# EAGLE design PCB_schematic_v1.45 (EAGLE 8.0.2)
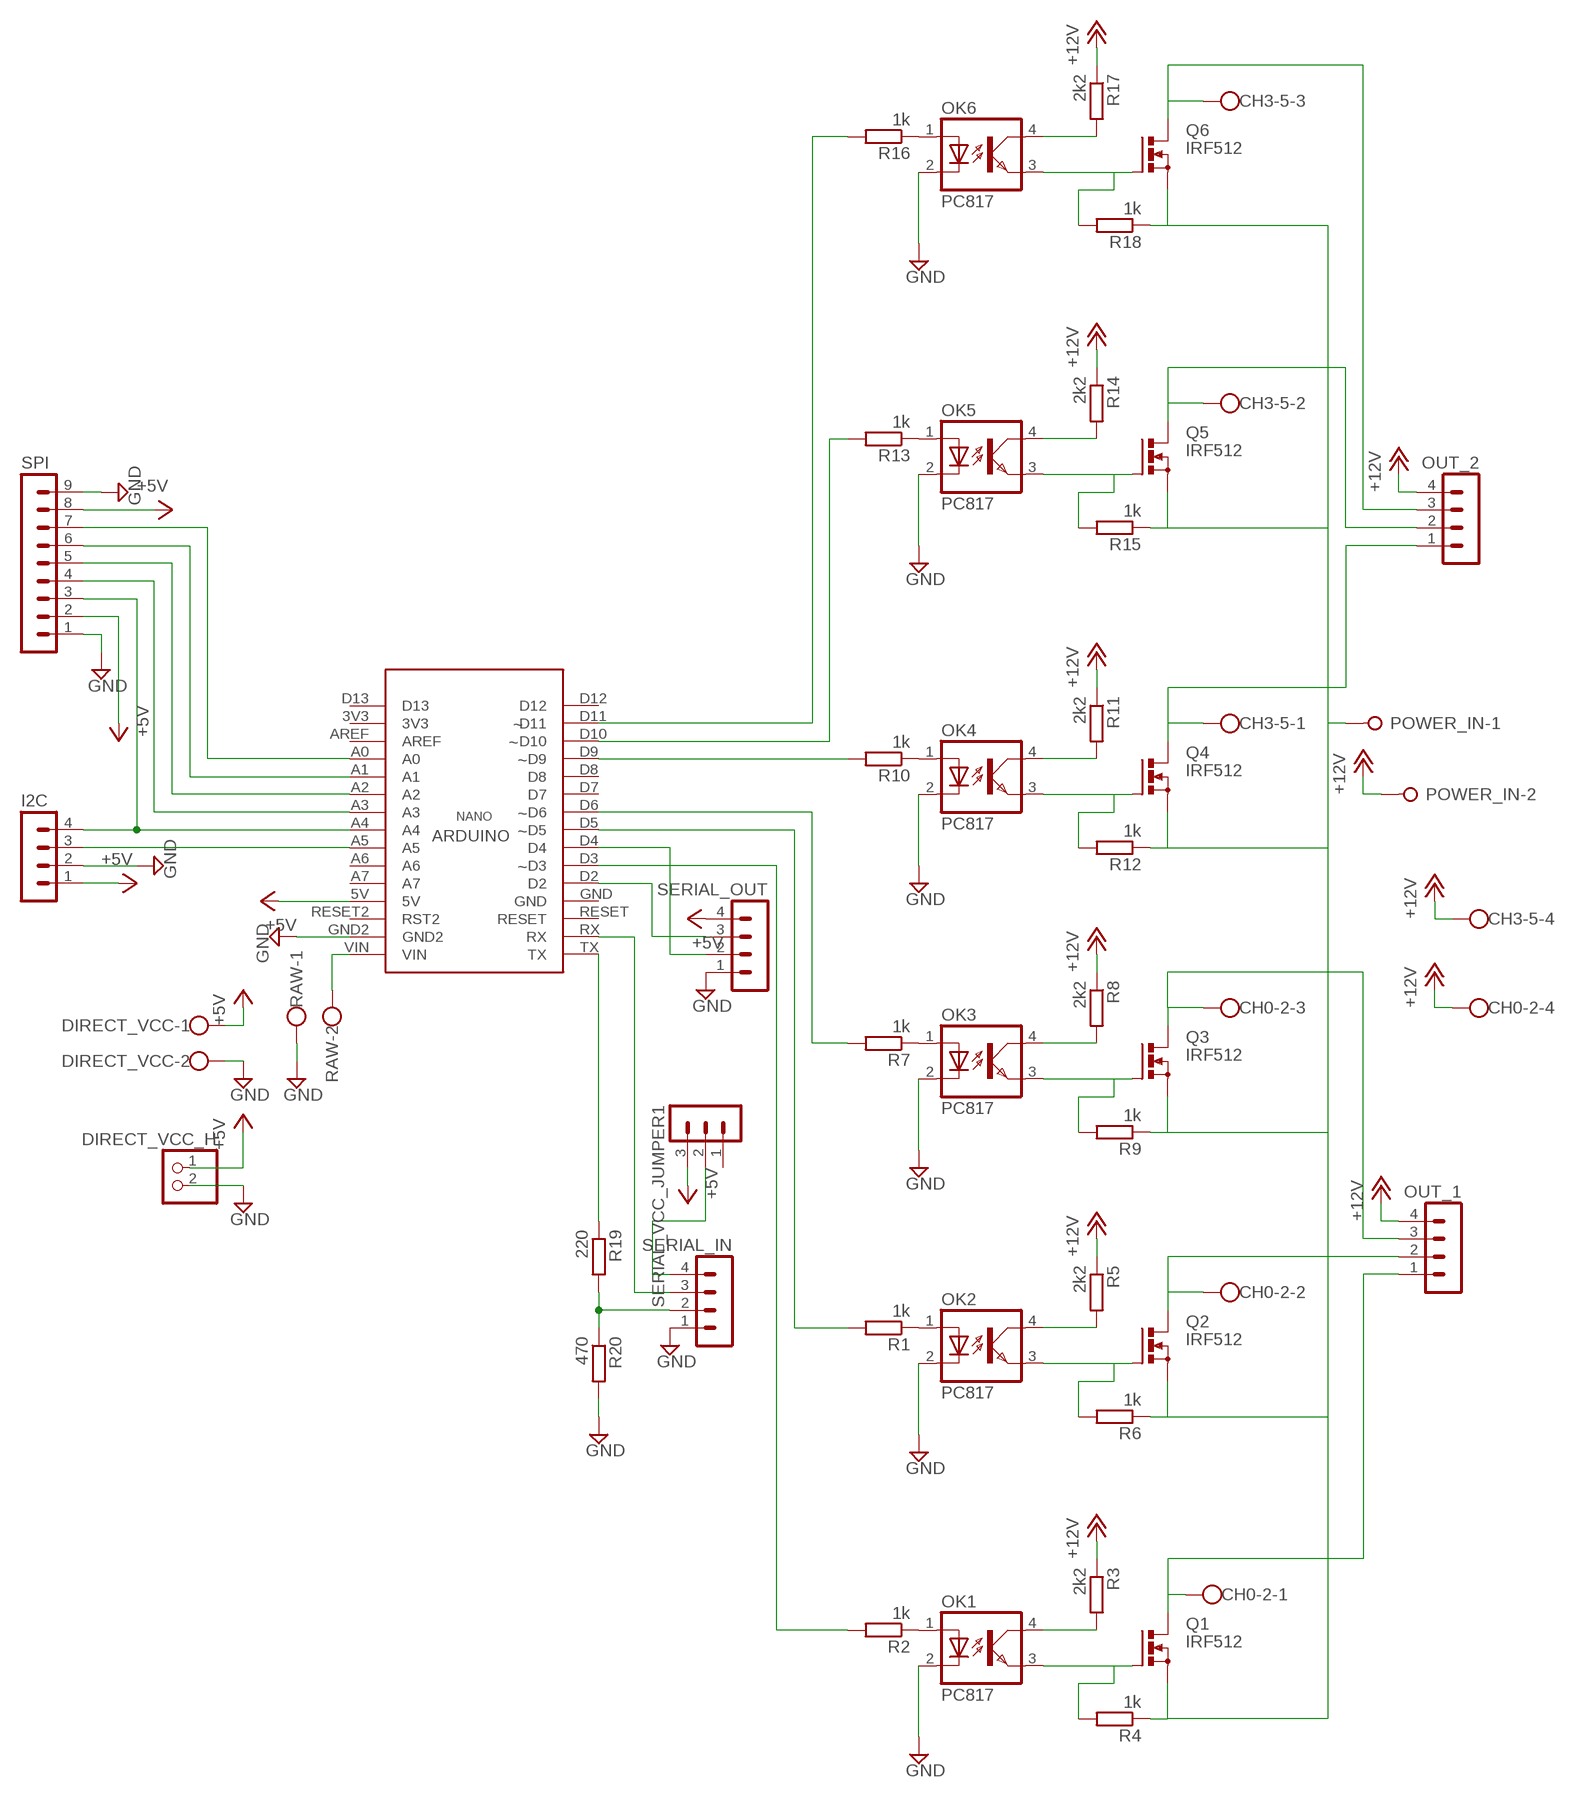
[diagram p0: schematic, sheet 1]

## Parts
CH0-2  W237-4  [W237-4]
CH3-5  W237-4  [W237-4]
DIRECT_VCC  W237-102  [W237-102]
DIRECT_VCC_H  PINHD-1X2  [1X02]
I2C  MA04-1  [MA04-1]
OK1  PC817  [DIL04]
OK2  PC817  [DIL04]
OK3  PC817  [DIL04]
OK4  PC817  [DIL04]
OK5  PC817  [DIL04]
OK6  PC817  [DIL04]
OUT_1  MA04-1  [MA04-1]
OUT_2  MA04-1  [MA04-1]
POWER_IN  W237-02P  [W237-132]
Q1  IRF512  [TO220BV]
Q2  IRF512  [TO220BV]
Q3  IRF512  [TO220BV]
Q4  IRF512  [TO220BV]
Q5  IRF512  [TO220BV]
Q6  IRF512  [TO220BV]
R1  1k  R-EU_0207/10  [0207/10]
R2  1k  R-EU_0207/10  [0207/10]
R3  2k2  R-EU_0207/10  [0207/10]
R4  1k  R-EU_0207/10  [0207/10]
R5  2k2  R-EU_0207/10  [0207/10]
R6  1k  R-EU_0207/10  [0207/10]
R7  1k  R-EU_0207/10  [0207/10]
R8  2k2  R-EU_0207/10  [0207/10]
R9  1k  R-EU_0207/10  [0207/10]
R10  1k  R-EU_0207/10  [0207/10]
R11  2k2  R-EU_0207/10  [0207/10]
R12  1k  R-EU_0207/10  [0207/10]
R13  1k  R-EU_0207/10  [0207/10]
R14  2k2  R-EU_0207/10  [0207/10]
R15  1k  R-EU_0207/10  [0207/10]
R16  1k  R-EU_0207/10  [0207/10]
R17  2k2  R-EU_0207/10  [0207/10]
R18  1k  R-EU_0207/10  [0207/10]
R19  220  R-EU_0207/10  [0207/10]
R20  470  R-EU_0207/10  [0207/10]
RAW  W237-102  [W237-102]
SERIAL_IN  MA04-1  [MA04-1]
SERIAL_OUT  MA04-1  [MA04-1]
SERIAL_VCC_JUMPER1  MA03-1  [MA03-1]
SPI  MA09-1  [MA09-1]
U$2  NANO  [NANO]

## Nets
+5V: DIRECT_VCC.1 DIRECT_VCC_H.1 I2C.1 SERIAL_OUT.4 SERIAL_VCC_JUMPER1.3 SPI.2 SPI.8 U$2.5V
+12V: CH0-2.4 CH3-5.4 OUT_1.4 OUT_2.4 POWER_IN.2 R3.1 R5.1 R8.1 R11.1 R14.1 R17.1
CS: SPI.7 U$2.A0
D1: SPI.4 U$2.A3
DC: SPI.6 U$2.A1
EXT_GND: POWER_IN.1 Q1.S Q2.S Q3.S Q4.S Q5.S Q6.S R4.1 R6.1 R9.1 R12.1 R15.1 R18.1
FET0_GATE: OK1.3(EMIT) Q1.G R4.2
FET0_GATE1: OK2.3(EMIT) Q2.G R6.2
FET0_GATE2: OK3.3(EMIT) Q3.G R9.2
FET0_GATE3: OK4.3(EMIT) Q4.G R12.2
FET0_GATE4: OK5.3(EMIT) Q5.G R15.2
FET0_GATE5: OK6.3(EMIT) Q6.G R18.2
GND: DIRECT_VCC.2 DIRECT_VCC_H.2 I2C.2 OK1.2(C) OK2.2(C) OK3.2(C) OK4.2(C) OK5.2(C) OK6.2(C) R20.2 RAW.1 SERIAL_IN.1 SERIAL_OUT.1 SPI.1 SPI.9 U$2.GND2
IC_PWM_OUT_0: R2.2 U$2.D3
IC_PWM_OUT_0_BASE: OK1.1(A) R2.1
IC_PWM_OUT_0_BASE1: OK2.1(A) R1.1
IC_PWM_OUT_0_BASE2: OK3.1(A) R7.1
IC_PWM_OUT_0_BASE3: OK4.1(A) R10.1
IC_PWM_OUT_0_BASE4: OK5.1(A) R13.1
IC_PWM_OUT_0_BASE5: OK6.1(A) R16.1
IC_PWM_OUT_1: R1.2 U$2.D5
IC_PWM_OUT_2: R7.2 U$2.D6
IC_PWM_OUT_3: R10.2 U$2.D9
IC_PWM_OUT_4: R13.2 U$2.D10
IC_PWM_OUT_5: R16.2 U$2.D11
N$1: OK1.4(COL) R3.2
N$3: OK2.4(COL) R5.2
N$5: OK3.4(COL) R8.2
N$7: OK4.4(COL) R11.2
N$9: OK5.4(COL) R14.2
N$11: OK6.4(COL) R17.2
OLED_RES: SPI.5 U$2.A2
OUT_RX: SERIAL_OUT.3 U$2.D2
OUT_TX: SERIAL_OUT.2 U$2.D4
OUTPUT_0: CH0-2.1 OUT_1.1 Q1.D
OUTPUT_1: CH0-2.2 OUT_1.2 Q2.D
OUTPUT_2: CH0-2.3 OUT_1.3 Q3.D
OUTPUT_3: CH3-5.1 OUT_2.1 Q4.D
OUTPUT_4: CH3-5.2 OUT_2.2 Q5.D
OUTPUT_5: CH3-5.3 OUT_2.3 Q6.D
RAW_INPUT: RAW.2 U$2.VIN
RX: SERIAL_IN.3 U$2.RX
SCL: I2C.3 U$2.A5
SDA_/_D0: I2C.4 SPI.3 U$2.A4
SERIAL_VCC: SERIAL_IN.4 SERIAL_VCC_JUMPER1.2
TX_3,3V: R19.2 R20.1 SERIAL_IN.2
TX_5V: R19.1 U$2.TX
Unconnected: SERIAL_VCC_JUMPER1.1 U$2.3V3 U$2.A6 U$2.A7 U$2.AREF U$2.D7 U$2.D8 U$2.D12 U$2.D13 U$2.GND U$2.RESET U$2.RESET2(RST2)

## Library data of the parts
CH0-2 CH3-5 = con-wago-500:W237-4: WAGO SCREW CLAMP; OC_FARNELL: unknown; OC_NEWARK: unknown
DIRECT_VCC RAW = con-wago-500:W237-102: WAGO SCREW CLAMP; MPN: 237-102; OC_FARNELL: unknown; OC_NEWARK: 70K9898
DIRECT_VCC_H = pinhead:PINHD-1X2: PIN HEADER
I2C OUT_1 OUT_2 SERIAL_IN SERIAL_OUT = con-lstb:MA04-1: PIN HEADER; OC_FARNELL: unknown; OC_NEWARK: unknown
OK1-OK6 = optocoupler:PC817: SHARP OPTO COUPLER; MPN: PC817X4J000F; OC_FARNELL: 9707727; OC_NEWARK: 97K7059
POWER_IN = con-wago-508:W237-02P: WAGO SREW CLAMP; OC_FARNELL: unknown; OC_NEWARK: unknown
Q1-Q6 = transistor-power:IRF512: N-CHANNEL MOS FET
R1-R20 = rcl:R-EU_: RESISTOR, European symbol
SERIAL_VCC_JUMPER1 = con-lstb:MA03-1: PIN HEADER; OC_FARNELL: unknown; OC_NEWARK: unknown
SPI = con-lstb:MA09-1: PIN HEADER; OC_FARNELL: unknown; OC_NEWARK: unknown
U$2 = NANO:NANO

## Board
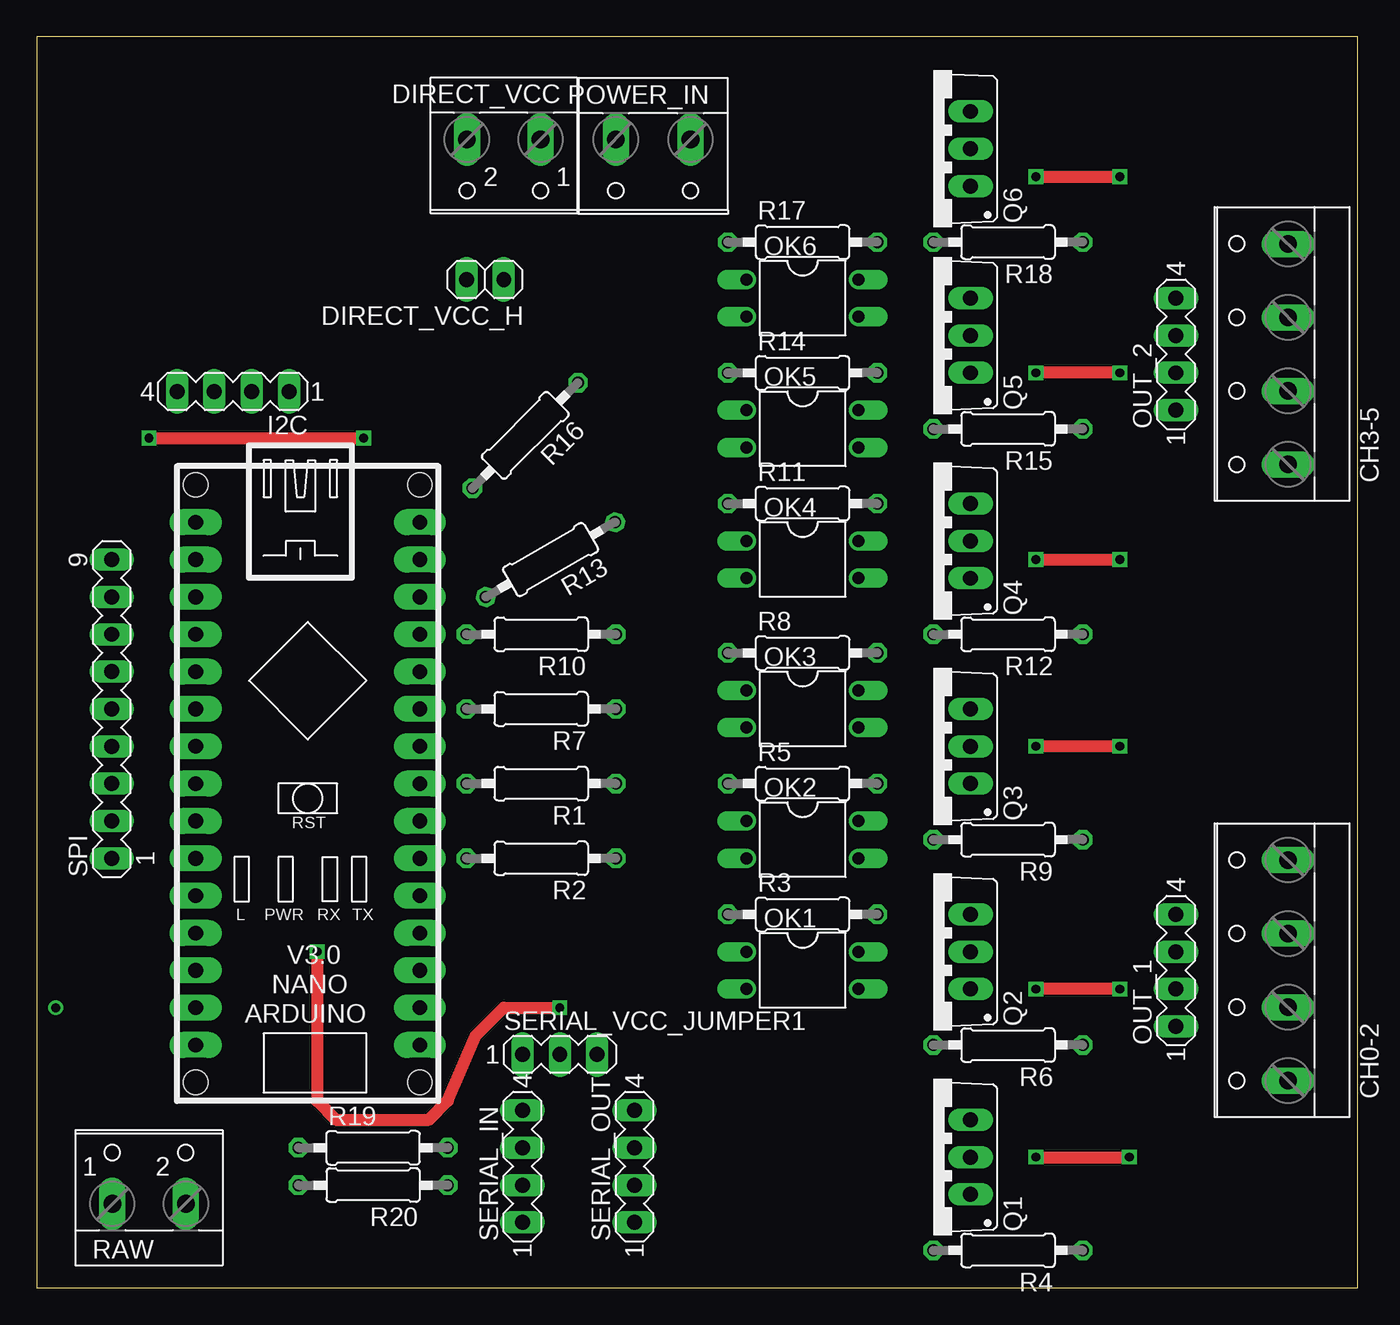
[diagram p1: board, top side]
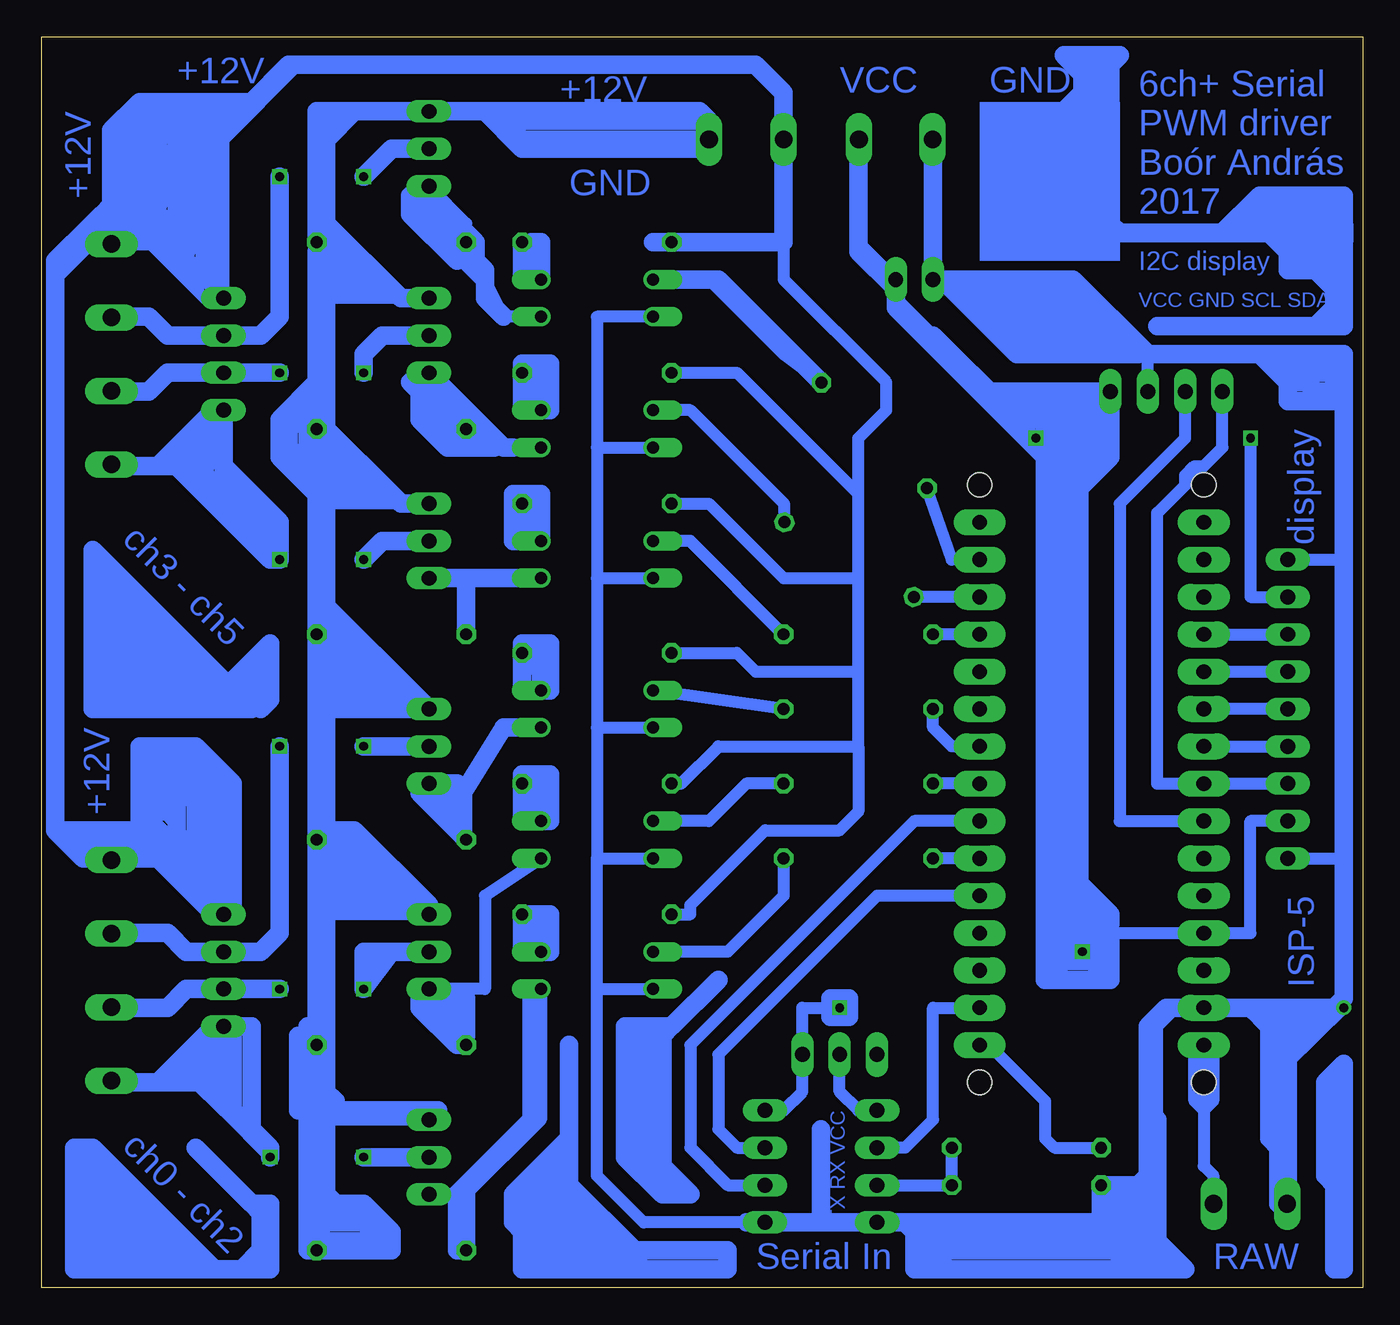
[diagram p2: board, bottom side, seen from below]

Size 89.84 x 85.08 mm. Coordinates in mm from the lower left corner, seen from the top.
Outline: 0,0 89.84,0 89.84,85.08 0,85.08 0,0
Copper layers (1*16): Top 0.035mm / dielectric 1.5mm / Bottom 0.035mm
Design rules "default": minimum track width 10mil, minimum drill 24mil, track to track 8mil, track to pad 8mil, pad to pad 8mil, via to via 8mil, smd to smd 8mil, copper to edge 40mil, drill to drill 8mil, minimum pad ring 10mil, minimum via ring 8mil, stop-mask expansion 4mil, vias tented up to drill 0mil, thermal gap 10mil

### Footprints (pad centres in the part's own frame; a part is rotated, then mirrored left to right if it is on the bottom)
W237-4 = drill 1.194 long: 1 -7.5,-1.27; 2 -2.5,-1.27; 3 2.5,-1.27; 4 7.5,-1.27
W237-102 = drill 1.194 long: 1 -2.5,-1.27; 2 2.5,-1.27
1X02 = drill 1.016 long: 1 -1.27,0; 2 1.27,0
MA04-1 = drill 1.016 long: 1 -3.81,0; 2 -1.27,0; 3 1.27,0; 4 3.81,0
DIL04 = drill 0.813 offset: 1 -1.27,-3.81; 2 1.27,-3.81; 3 1.27,3.81; 4 -1.27,3.81
W237-132 = drill 1.194 long: 1 -2.54,-0.635; 2 2.54,-0.635
TO220BV = drill 1.016 long: D 0,-2.54; G -2.54,-2.54; S 2.54,-2.54
0207/10 = drill 0.813 octagon: 1 -5.08,0; 2 5.08,0
MA03-1 = drill 1.016 long: 1 -2.54,0; 2 0,0; 3 2.54,0
MA09-1 = drill 1.016 long: 1 -10.16,0; 2 -7.62,0; 3 -5.08,0; 4 -2.54,0; 5 0,0; 6 2.54,0; 7 5.08,0; 8 7.62,0; 9 10.16,0
NANO = drill 1 pad 1.778 long: 3V3 7.62,-15.24; 5V 7.62,10.16; A0 7.62,-10.16; A1 7.62,-7.62; A2 7.62,-5.08; A3 7.62,-2.54; A4 7.62,0; A5 7.62,2.54; A6 7.62,5.08; A7 7.62,7.62; AREF 7.62,-12.7; D2 -7.62,7.62; D3 -7.62,5.08; D4 -7.62,2.54; D5 -7.62,0; D6 -7.62,-2.54; D7 -7.62,-5.08; D8 -7.62,-7.62; D9 -7.62,-10.16; D10 -7.62,-12.7; D11 -7.62,-15.24; D12 -7.62,-17.78; D13 7.62,-17.78; GND -7.62,10.16; GND2 7.62,15.24; RESET -7.62,12.7; RESET2 7.62,12.7; RX -7.62,15.24; TX -7.62,17.78; VIN 7.62,17.78 | hole 1.651: -7.62,-20.32; 7.62,-20.32; -7.62,20.32; 7.62,20.32

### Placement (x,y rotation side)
CH0-2  83.82,21.59 90 top
CH3-5  83.82,63.5 90 top
DIRECT_VCC  31.75,76.83 180 top
DIRECT_VCC_H  30.48,68.58 180 top
I2C  13.34,60.96 180 top
OK1  52.07,21.59 270 top
OK2  52.07,30.48 270 top
OK3  52.07,39.37 270 top
OK4  52.07,49.53 270 top
OK5  52.07,58.42 270 top
OK6  52.07,67.31 270 top
OUT_1  77.47,21.59 90 top
OUT_2  77.47,63.5 90 top
POWER_IN  41.91,77.47 180 top
Q1  60.96,8.89 90 top
Q2  60.96,22.86 90 top
Q3  60.96,36.83 90 top
Q4  60.96,50.8 90 top
Q5  60.96,64.77 90 top
Q6  60.96,77.47 90 top
R1  34.29,34.29 180 top
R2  34.29,29.21 180 top
R3  52.07,25.4 0 top
R4  66.04,2.54 180 top
R5  52.07,34.29 0 top
R6  66.04,16.51 180 top
R7  34.29,39.37 180 top
R8  52.07,43.18 0 top
R9  66.04,30.48 180 top
R10  34.29,44.45 180 top
R11  52.07,53.34 0 top
R12  66.04,44.45 180 top
R13  34.92,49.53 210 top
R14  52.07,62.23 0 top
R15  66.04,58.42 180 top
R16  33.21,57.97 225 top
R17  52.07,71.12 0 top
R18  66.04,71.12 180 top
R19  22.86,9.53 0 top
R20  22.86,6.99 180 top
RAW  7.62,6.99 0 top
SERIAL_IN  33.02,8.26 90 top
SERIAL_OUT  40.64,8.26 90 top
SERIAL_VCC_JUMPER1  35.56,15.88 0 top
SPI  5.08,39.37 90 top
U$2  18.41,34.29 180 top

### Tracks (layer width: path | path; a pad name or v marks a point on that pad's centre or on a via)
+5V  (via drill 0.6)
  Top 0.813: v7.62,57.78 v22.23,57.78 | v19.05,22.86 19.05,12.7 20.32,11.43 26.67,11.43 27.94,12.7 29.84,17.14 31.75,19.05 v35.56,19.05
  Bottom 0.813: DIRECT_VCC.1 34.25,71.08 DIRECT_VCC_H.1 31.75,67.31 24.13,59.69 v22.23,57.78 | 19.05,25.4 19.05,27.3 19.05,54.61 21.59,57.15 v22.23,57.78 | 19.05,25.4 17.78,24.13 17.14,24.13 U$2.5V 7.62,24.13 7.62,31.75 SPI.2 | v7.62,57.78 7.62,46.99 SPI.8 | 19.05,25.4 v19.05,22.86 | I2C.1 17.14,59.05 20.95,59.05 v22.23,57.78 | v35.56,19.05 38.1,19.05 SERIAL_VCC_JUMPER1.3 38.1,13.34 39.37,12.06 SERIAL_OUT.4
  Bottom 1.27: 17.14,24.13 17.14,22.23 | 17.14,22.23 18.41,20.95 | 18.41,20.95 20.32,20.95 | 20.32,20.95 21.59,22.23 21.59,22.86 20.95,23.5 | 20.95,23.5 19.68,24.77 19.68,58.42 18.41,58.42 | 18.41,58.42 18.41,55.24 | 18.41,55.24 19.05,54.61 19.05,57.15 20.32,58.42 20.95,58.42 21.59,57.78 | 20.95,57.78 20.32,57.15 20.32,56.52 20.95,57.15 21.59,57.78 | 20.95,23.5 20.95,55.88 26.04,60.96 | 20.95,23.5 20.95,22.86 | 20.95,22.86 20.32,22.23 18.41,22.23 18.41,24.13 19.05,24.13 20.32,22.86 | 17.14,24.77 17.14,25.4 19.05,27.3 19.05,26.67 17.78,25.4 | 17.78,24.77 17.78,24.13 17.78,22.86 17.14,22.23 | 17.14,22.23 17.14,20.95 18.41,20.95 | 20.32,20.95 20.95,20.95 | 20.95,20.95 20.95,22.86 | v35.56,19.05 34.92,19.68 | v35.56,19.05 36.2,18.41 | 36.2,18.41 36.2,19.68 34.92,19.68 | 34.92,19.68 34.92,18.41 | 29.84,64.77 31.75,66.67 31.75,67.94 34.29,70.48 34.29,78.11 | 36.2,18.41 34.92,18.41 | 34.92,18.41 v35.56,19.05 | 20.95,20.95 21.59,20.95 21.59,57.15 | 20.95,59.05 19.05,59.05 I2C.1 | I2C.1 17.14,56.52 18.41,55.24 | 18.41,58.42 18.41,59.69 I2C.1 | I2C.1 26.04,60.96 | 26.04,60.96 29.84,64.77 | 29.84,64.77 29.21,64.77 24.13,59.69 19.05,59.69 18.41,60.33 21.59,60.33 22.86,59.05 21.59,59.05 21.59,57.78
+12V
  Bottom 0.813: 72.39,83.19 77.47,78.11 OUT_2.4 78.74,67.31 82.43,71 CH3-5.4 85.21,71.12 86.36,71.12 88.9,68.58 88.9,31.11 | 39.37,81.28 POWER_IN.2 39.37,71.12 39.37,68.58 32.38,61.59 32.38,59.69 34.29,57.78 34.29,53.98 | R3.1 45.72,25.4 45.72,26.04 40.64,31.11 35.56,31.11 34.29,32.38 34.29,36.83 | 34.29,48.26 34.29,53.98 | 34.29,41.91 34.29,48.26 | 34.29,36.83 34.29,41.91 | R14.1 42.55,62.23 34.29,53.98 | R11.1 44.45,53.34 39.37,48.26 34.29,48.26 | R8.1 42.55,43.18 41.27,41.91 34.29,41.91 | R5.1 46.35,34.29 43.81,36.83 34.29,36.83 | OUT_1.4 81.16,29.09 CH0-2.4 86.88,29.09 87,29.21
  Bottom 1.27: 78.11,67.94 78.11,78.11 75.56,80.64 | 76.2,80.64 83.19,80.64 85.09,78.74 85.09,73.66 85.72,73.03 | 86.36,72.39 88.9,69.85 88.9,31.11 87,29.21 81.92,29.21 78.11,25.4 76.83,25.4 76.83,34.29 79.38,36.83 83.19,36.83 83.19,35.56 | 86.36,72.39 83.82,72.39 83.19,71.75 81.92,71.75 78.74,68.58 78.74,78.74 77.47,80.01 82.55,80.01 84.45,78.11 84.45,73.66 83.82,73.03 82.55,73.03 80.01,70.48 80.01,78.74 79.38,79.38 81.92,79.38 83.82,77.47 83.82,73.66 82.55,73.66 80.64,71.75 80.64,78.11 81.28,78.74 82.55,77.47 82.55,76.2 83.19,75.56 83.19,74.93 | 83.19,74.93 81.92,73.66 81.92,74.93 | 81.92,74.93 81.28,75.56 81.28,76.83 81.92,77.47 81.92,74.93 | 81.92,74.93 83.19,74.93 | 83.19,74.93 85.09,73.03 85.72,73.03 | 85.72,73.03 86.36,72.39 | 83.19,32.38 83.19,31.11 87.63,31.11 | 88.27,31.11 87.63,31.11 | 87.63,31.11 86.36,29.84 83.82,29.84 83.19,30.48 82.55,30.48 | 82.55,30.48 81.28,30.48 | 81.28,30.48 77.47,26.67 77.47,33.66 80.01,36.2 82.55,36.2 83.19,35.56 | 83.19,35.56 83.19,32.38 | 83.19,32.38 81.28,30.48 | 81.28,30.48 80.64,30.48 | 80.64,30.48 80.01,30.48 78.11,28.57 78.11,33.02 78.74,33.66 79.38,33.66 81.28,35.56 80.64,35.56 79.38,34.29 79.38,31.11 78.74,30.48 78.74,32.38 81.92,35.56 81.92,33.66 82.55,33.02 82.55,32.38 81.28,32.38 80.64,31.75 | 80.64,31.75 80.64,32.38 | 80.64,32.38 80.64,33.66 81.28,34.29 81.28,33.02 80.64,32.38 | 80.64,31.75 80.64,30.48 | 81.28,29.84 82.55,29.84 82.55,30.48 | 75.56,80.64 73.03,83.19 72.39,83.19 41.27,83.19 39.37,81.28 39.37,71.12 R17.1 48.26,71.12 | 75.56,80.64 76.2,80.64 | 76.2,80.64 78.11,78.74
CS
  Bottom 0.813: U$2.A0 SPI.7
D1
  Bottom 0.813: U$2.A3 SPI.4
DC
  Bottom 0.813: U$2.A1 SPI.6
EXT_GND
  Bottom 0.813: 71.12,11.43 71.12,6.99 71.12,5.71 R4.1 | 71.12,11.43 R6.1 71.12,17.78 71.12,25.4 | 71.12,25.4 71.12,26.04 | 71.12,39.37 71.12,31.11 R9.1 | 71.12,39.37 71.12,40.01 | 71.12,41.27 R12.1 71.12,46.99 | 71.12,53.34 71.12,55.24 R15.1 71.12,61.59 71.12,67.31 | 71.12,53.34 71.12,47.62 | Q5.S 64.14,67.31 71.12,67.31 | Q4.S 71.12,53.34 | Q2.S 71.12,25.4 | Q1.S 70.48,11.43 71.12,11.43 | 59.69,80.01 Q6.S 67.94,80.01 71.12,80.01 | R18.1 71.12,70.48 71.12,67.31 | Q3.S 71.12,39.37
  Bottom 1.27: 71.12,31.11 68.58,31.11 63.5,26.04 71.12,26.04 R9.1 69.22,30.48 65.41,26.67 67.31,26.67 | 69.22,26.67 69.85,26.67 69.85,27.3 | 69.85,27.3 69.85,29.21 | 69.85,29.21 70.48,29.84 | 69.85,29.21 67.31,26.67 | 67.31,26.67 69.22,26.67 | 69.22,26.67 69.85,27.3 | 69.85,29.21 69.85,29.84 67.31,27.3 69.85,27.3 | 71.12,46.99 71.12,47.62 71.12,53.98 73.66,56.52 73.66,59.05 | 71.12,46.99 Q3.S 70.48,39.37 71.12,40.01 | 71.12,46.35 71.12,41.27 71.12,17.78 71.75,17.78 | 71.12,46.99 71.12,46.35 | 71.12,46.35 64.77,40.01 66.04,40.01 | 69.22,40.01 70.48,40.01 70.48,44.45 | 70.48,45.09 70.48,44.45 | 70.48,44.45 66.04,40.01 | 66.04,40.01 69.22,40.01 | 69.22,40.01 69.85,40.64 69.85,42.55 67.94,40.64 69.22,40.64 | Q4.S 65.41,53.34 66.04,53.98 | 66.04,53.98 70.48,58.42 | 70.48,58.42 70.48,57.15 | 70.48,57.15 70.48,53.98 67.31,53.98 | 66.04,53.98 67.31,53.98 | 67.31,53.98 69.85,56.52 69.85,55.24 69.22,54.61 | 64.14,67.31 65.41,67.31 70.48,72.39 70.48,67.94 67.31,67.94 69.85,70.48 69.85,68.58 68.58,68.58 | 71.75,11.43 71.75,2.54 R4.1 66.04,2.54 66.04,3.81 67.94,5.71 69.85,5.71 | 69.85,5.71 70.48,5.71 | 70.48,5.71 71.12,5.71 71.12,3.81 70.48,3.17 66.67,3.17 67.94,4.45 70.48,4.45 | 69.85,5.71 71.12,6.99 71.12,10.79 70.48,11.43 | 73.66,59.05 71.75,59.69 | 71.75,59.69 71.75,55.88 | 71.75,55.88 71.12,55.24 | 71.75,55.88 73.03,57.15 73.03,58.42 72.39,59.05 | 71.75,59.69 70.48,58.42 | 73.66,59.05 71.12,61.59 | 71.12,61.59 71.12,70.48 | 71.12,61.59 71.12,57.78 70.48,57.15 | R18.1 71.12,77.47 | 71.12,78.74 71.12,80.01 68.58,80.01 | 59.69,80.01 67.94,80.01 68.58,80.01 | 59.69,80.01 59.05,80.01 | 59.05,80.01 57.15,78.11 POWER_IN.1 | 44.45,77.47 57.15,77.47 59.69,80.01
  Bottom 1.27: 59.05,80.01 45.09,80.01 44.45,79.38 57.15,79.38 | 68.58,80.01 70.48,78.11 | 70.48,78.11 71.12,77.47 | 71.12,77.47 71.12,78.74 | 71.12,78.74 70.48,79.38 | 70.48,78.11 70.48,5.71
FET0_GATE
  Bottom 0.813: R4.2 60.96,6.35 | OK1.3 55.88,11.43 60.96,6.35 | 60.96,6.35 61.59,6.35 Q1.G
  Bottom 1.27: 56.52,19.68 56.52,11.43 60.96,6.99 | 60.96,6.99 61.59,6.35 61.59,2.54 R4.2 60.96,6.99
FET0_GATE1
  Bottom 0.813: R6.2 60.96,17.14 | 60.96,19.68 60.96,20.32 | OK2.3 59.69,26.67 59.69,20.32 60.96,20.32 | 60.96,20.32 Q2.G
  Bottom 1.27: R6.2 61.59,16.51 64.14,19.05 64.14,20.32 60.96,17.14 60.96,19.68 62.23,19.68 61.59,19.05
FET0_GATE2
  Bottom 0.813: 60.96,34.29 61.59,34.29 Q3.G | 58.42,38.1 60.96,34.29 | 60.96,34.29 R9.2
  Bottom 1.27: R9.2 64.14,33.66 64.14,34.29 61.59,34.29 61.59,33.02 | 61.59,33.02 61.59,32.38 62.23,32.38 63.5,33.66 62.23,33.66 61.59,33.02 | 61.59,33.02 58.42,38.1 OK3.3
FET0_GATE3
  Bottom 0.813: OK4.3 60.96,48.26
  Bottom 1.27: R12.2 60.96,48.26 Q4.G OK4.3
FET0_GATE4
  Bottom 0.813: Q5.G 62.87,61.59 60.96,59.69 R15.2 59.69,58.42 58.42,57.15 | OK5.3 57.78,57.15
  Bottom 1.27: 60.33,59.05 60.96,59.69 61.59,59.05 | 61.59,59.05 62.23,58.42 62.23,57.15 | 62.23,57.15 59.69,57.15 | 59.05,57.15 59.69,57.15 | 59.69,57.15 R15.2 61.59,57.78 | 62.23,57.15 64.14,59.05 64.14,60.96 64.77,61.59 63.5,61.59 62.87,60.96 62.87,60.33 61.59,59.05 | 61.59,59.05 62.87,59.05 63.5,59.69 63.5,60.33 61.59,60.33 | 61.59,60.33 58.42,57.15 57.78,57.15 | 61.59,60.33 62.87,61.59
FET0_GATE5
  Bottom 0.813: Q6.G 60.96,72.39 R18.2 60.33,69.85 59.69,68.58 58.42,66.04 OK6.3
  Bottom 1.27: 58.42,66.04 59.69,67.31 59.69,68.58 | 60.33,69.22 60.96,69.85 60.96,70.48 | 60.96,70.48 R18.2 60.33,71.12 | 60.33,69.85 60.33,69.22 | 60.33,69.22 59.69,68.58 | 59.69,68.58 59.69,69.22 60.33,69.85 | 60.33,69.85 60.33,71.12 | 60.33,71.12 63.5,74.3 | 61.59,69.85 64.77,73.03 64.77,74.3 60.96,70.48
GND  (via drill 0.6)
  Bottom 0.813: OK6.2 52.07,66.04 52.07,57.15 | 52.07,57.15 OK5.2 | 52.07,57.15 52.07,48.26 | 52.07,48.26 OK4.2 | 52.07,48.26 52.07,38.1 | 52.07,38.1 OK3.2 | 52.07,38.1 52.07,29.21 | 52.07,29.21 OK2.2 | 52.07,20.32 52.07,29.21 | 52.07,20.32 OK1.2 | 52.07,20.32 52.07,7.62 48.9,4.45 41.91,4.45 SERIAL_OUT.1 36.83,4.45 SERIAL_IN.1 24.77,4.45 | R20.2 17.14,4.45 | 17.14,4.45 14.61,6.99 13.97,7.62 13.97,17.78 12.7,19.05 U$2.GND2 7.62,19.05 | 1.27,49.53 1.27,29.21 | 1.27,49.53 1.27,60.33 | v1.27,19.05 1.27,29.21 | v1.27,19.05 5.12,15.28 RAW.1 | SPI.1 1.27,29.21 | SPI.9 1.27,49.53 | DIRECT_VCC.2 29.25,68.62 DIRECT_VCC_H.2 | 17.14,4.45 17.78,4.45 | I2C.2 14.61,63.5 | 1.91,19.05 v1.27,19.05
  Bottom 1.27: 29.21,78.11 DIRECT_VCC_H.2 28.57,68.58 | 20.95,68.58 19.68,68.58 14.61,63.5 6.99,63.5 | 6.35,63.5 1.27,63.5 1.27,60.33 | 1.27,60.33 1.27,19.68 1.91,19.05 | 1.91,19.05 2.54,18.41 | 2.54,18.41 5.08,15.88 5.08,6.35 5.71,5.71 5.71,9.53 6.35,10.16 6.35,17.78 6.99,18.41 | 6.99,18.41 3.81,18.41 | 2.54,18.41 3.81,18.41 | 3.81,18.41 5.71,16.51 5.71,17.78 | R20.2 17.78,4.45 24.77,4.45 | 24.77,4.45 25.4,3.81 27.94,3.81 29.21,2.54 | 29.21,1.27 15.24,1.27 | 13.34,1.27 12.06,1.27 13.97,3.17 13.97,4.45 | 14.61,3.81 16.51,1.91 15.88,1.91 | 15.88,1.91 14.61,1.91 13.97,2.54 14.61,2.54 13.34,1.27 | 13.34,1.27 15.24,1.27 | 15.24,1.27 15.88,1.91 | 15.88,1.91 15.24,2.54 25.4,2.54 | 29.21,2.54 30.48,1.27 | 30.48,1.27 29.21,1.27 | 29.21,1.27 28.57,1.91 | 29.21,2.54 25.4,2.54 | 25.4,2.54 24.13,3.81 17.14,3.81 | 17.14,3.81 14.61,3.81 | 14.61,3.81 13.97,4.45 | 13.97,4.45 13.97,11.43 14.61,12.06 | 14.61,12.06 14.61,17.78 13.34,19.05 7.62,19.05 | 6.99,18.41 7.62,19.05 | 7.62,19.05 1.91,19.05 | 17.14,3.81 14.61,6.35 14.61,5.08 15.24,4.45 R20.2 | R20.2 15.88,6.99 | 14.61,6.99 15.88,6.99 | 15.88,6.99 16.51,6.35 15.88,6.35 14.61,7.62 14.61,12.06 | 36.83,10.79 36.83,4.45 | 31.11,4.45 24.77,4.45 | 36.83,4.45 41.91,4.45 | 36.83,4.45 31.11,4.45 | 31.11,4.45 30.48,3.81 30.48,2.54 | 30.48,1.27 30.48,2.54 | 30.48,2.54 29.21,3.81 | 15.24,63.5 23.5,63.5 28.57,68.58 | 28.57,68.58 20.95,68.58 | 20.95,68.58 16.51,64.14 22.86,64.14 26.67,67.94 21.59,67.94 18.41,64.77 22.23,64.77 24.77,67.31 22.23,67.31 20.32,65.41 21.59,65.41 22.86,66.67 | 1.27,60.33 5.08,60.33 5.08,61.59 6.99,63.5 | 6.99,63.5 6.35,63.5 | 6.35,63.5 4.45,61.59 3.81,61.59 3.17,60.96 1.91,60.96 1.91,62.23 3.81,62.23 4.45,62.87
IC_PWM_OUT_0
  Bottom 0.813: U$2.D3 R2.2
IC_PWM_OUT_0_BASE
  Bottom 0.813: R2.1 39.37,26.67 43.18,22.86 OK1.1
IC_PWM_OUT_0_BASE1
  Bottom 0.813: R1.1 41.91,34.29 44.45,31.75 OK2.1
IC_PWM_OUT_0_BASE2
  Bottom 0.813: R7.1 OK3.1
IC_PWM_OUT_0_BASE3
  Bottom 0.813: R10.1 45.72,50.8 OK4.1
IC_PWM_OUT_0_BASE4
  Bottom 0.813: OK5.1 45.72,59.69 39.32,53.29 R13.1
IC_PWM_OUT_0_BASE5
  Bottom 0.813: R16.1 39.37,63.5 44.45,68.58 OK6.1
  Bottom 1.27: 36.83,61.59 43.81,68.58 OK6.1
IC_PWM_OUT_1
  Bottom 0.813: U$2.D5 R1.2
IC_PWM_OUT_2
  Bottom 0.813: U$2.D6 27.94,36.83 29.21,38.1 R7.2
IC_PWM_OUT_3
  Bottom 0.813: U$2.D9 R10.2
IC_PWM_OUT_4
  Bottom 0.813: U$2.D10 R13.2
IC_PWM_OUT_5
  Bottom 0.813: R16.2 27.94,49.53 U$2.D11
N$1
  Bottom 0.813: OK1.4 55.88,24.13 R3.2
  Bottom 1.27: 57.15,22.86 R3.2 55.24,25.4 55.24,22.86 56.52,22.86 56.52,24.13
N$2
  Bottom 1.27: 10.16,71.75 9.53,71.75 6.99,74.3 1.27,74.3 | 1.27,74.3 1.27,69.85 | 1.27,68.58 1.27,67.31 | 1.27,66.67 1.27,65.41 3.17,65.41 | 13.97,65.41 3.17,65.41 | 3.17,65.41 1.27,67.31 | 1.27,67.31 1.27,66.67 | 1.27,66.67 1.91,66.04 1.91,67.94 3.17,69.22 5.08,69.22 5.08,70.48 | 5.08,70.48 6.99,72.39 7.62,72.39 | 5.08,70.48 4.45,69.85 2.54,69.85 1.27,68.58 | 1.27,68.58 1.27,69.85 | 1.27,69.85 2.54,71.12 4.45,71.12 5.08,70.48 | 8.26,72.39 7.62,72.39 | 7.62,72.39 6.35,73.66 1.91,73.66 1.91,73.03 2.54,72.39 5.71,72.39 6.35,73.03 2.54,73.03 1.27,74.3
N$3
  Bottom 0.813: OK2.4 55.88,33.02 56.52,33.66 R5.2
  Bottom 1.27: 57.15,33.02 57.15,34.92 55.24,34.92 55.24,31.75 57.15,31.75 57.15,33.02 | 57.15,33.02 56.52,33.66 | 56.52,32.38 56.52,33.66 | 56.52,33.66 55.88,34.29
N$4
  Bottom 1.27: 15.88,71.75 16.51,71.75 17.14,72.39 17.14,83.19 16.51,83.82 20.32,83.82 19.05,82.55 19.05,81.28 | 19.05,81.28 19.05,80.64 19.68,80.01 | 19.68,80.01 18.41,80.01 17.78,80.64 17.78,83.19 19.05,83.19 | 19.05,81.28 20.32,80.01 19.68,80.01
N$5
  Bottom 0.813: 56.52,42.55 R8.2
  Bottom 1.27: 57.15,40.64 57.15,43.81 55.24,43.81 55.24,40.64 OK3.4 55.88,41.91 56.52,42.55 56.52,43.18
N$6
  Bottom 1.27: 46.99,6.35 47.62,6.35 50.16,8.89 50.16,17.78 48.26,17.78 | 48.26,17.78 48.26,16.51 | 48.26,16.51 48.26,8.89 47.62,8.26 | 46.99,6.35 45.72,6.35 47.62,8.26 | 46.99,6.35 49.53,8.89 49.53,16.51 48.9,17.14 | 48.26,17.78 46.99,17.78 | 46.99,17.78 43.81,20.95 | 46.99,17.78 47.62,17.14 | 48.26,16.51 47.62,17.14 | 47.62,17.14 47.62,8.26
N$7
  Bottom 0.813: OK4.4 55.88,52.07 R11.2
  Bottom 1.27: OK4.4 55.88,53.98 57.78,53.98 57.78,50.8 56.52,50.8 56.52,52.07 57.15,52.7
N$9
  Bottom 0.813: OK5.4 55.88,60.96 R14.2
N$11
  Bottom 0.813: OK6.4 55.88,69.85 R17.2
  Bottom 1.27: 56.52,68.58 56.52,70.48 R17.2 57.15,68.58 OK6.4 55.88,71.12 56.52,71.12
N$24
  Bottom 1.27: 53.98,6.99 49.53,2.54 43.18,2.54 43.18,1.27 48.9,1.27 | 54.61,7.62 53.98,6.99 | 53.98,6.99 53.98,8.26 | 53.98,8.89 53.98,10.16 | 53.98,16.51 53.98,10.16 | 53.98,10.16 57.78,6.35 57.78,4.45 57.15,3.81 | 57.15,3.17 57.15,1.27 48.9,1.27 | 48.9,1.27 55.24,7.62 53.98,8.89 | 53.98,8.89 53.98,8.26 | 53.98,8.26 57.15,5.08 57.15,3.81 | 57.15,3.81 57.15,3.17 | 57.15,3.17 55.88,1.91 50.8,1.91 | 50.16,1.91 50.8,1.91 | 50.8,1.91 55.24,6.35 55.24,5.71 | 55.24,5.71 57.15,3.81 | 57.15,3.81 55.88,2.54 52.7,2.54 52.7,3.17 53.34,3.81 | 53.34,3.81 55.24,5.71 | 55.24,5.71 55.24,5.08 | 55.24,5.08 55.24,4.45 55.88,3.81 54.61,3.81 | 53.34,3.81 54.61,3.81 | 54.61,3.81 57.15,6.35 55.88,7.62 55.88,5.71 55.24,5.08
N$27
  Bottom 1.27: 1.27,1.27 1.27,15.24 2.54,13.97 2.54,7.62 1.91,6.99 1.91,1.27 1.27,1.27
N$28
  Bottom 1.27: 79.38,1.27 87,8.89 87.63,9.53 | 87.63,9.53 87.63,1.27 80.64,1.27 | 80.64,1.27 87,7.62 87,2.54 86.36,1.91 82.55,1.91 86.36,5.71 86.36,3.81 | 86.36,3.81 86.36,2.54 85.09,2.54 | 83.82,2.54 85.09,2.54 | 85.09,2.54 86.36,3.81 | 86.36,3.81 85.09,3.81 84.45,3.17 | 80.64,1.27 78.11,1.27 | 76.2,1.27 74.93,1.27 | 74.93,1.27 74.3,1.27 74.3,4.45 | 74.3,4.45 74.3,5.71 75.56,5.71 | 75.56,5.71 79.38,9.53 | 75.56,5.71 74.93,5.08 | 74.3,4.45 74.93,5.08 | 74.93,5.08 74.93,2.54 | 74.93,1.27 74.93,2.54 | 74.93,2.54 76.2,1.27 | 76.2,1.27 78.11,1.27 | 78.11,1.27 86.36,9.53 87.63,9.53
N$29
  Bottom 1.27: 62.87,12.06 72.39,12.06 72.39,17.14 70.48,17.14 70.48,13.34 69.85,12.7 71.75,12.7 71.75,16.51
N$31
  Bottom 1.27: 57.15,59.69 57.15,62.87 55.24,62.87 55.24,59.69 56.52,59.69 56.52,62.23
N$32
  Bottom 1.27: 75.56,39.37 86.36,39.37 86.36,50.16 77.47,41.27 76.83,41.27 74.3,43.81 74.3,40.01 74.93,39.37 74.93,41.91 76.2,40.64 75.56,40.01 84.45,40.01 85.09,40.64 85.09,47.62 85.72,48.26 85.72,40.64 85.09,40.01 78.74,40.01 78.11,40.64 84.45,46.99 84.45,41.27 83.82,40.64 79.38,40.64 83.82,45.09 83.82,43.18 | 83.82,43.18 83.82,41.91 83.19,41.27 81.92,41.27 | 80.64,41.27 81.92,41.27 | 81.92,41.27 83.82,43.18 | 83.82,43.18 82.55,43.18 81.28,41.91
OLED_RES
  Bottom 0.813: SPI.5 U$2.A2
OUT_RX
  Bottom 0.813: U$2.D2 33.02,26.67 43.81,15.88 43.81,10.79 42.55,9.53 SERIAL_OUT.3
OUT_TX
  Bottom 0.813: U$2.D4 30.48,31.75 45.72,16.51 45.72,9.53 43.18,6.99 SERIAL_OUT.2
OUTPUT_0  (via drill 0.6)
  Top 0.813: v67.94,8.89 v74.3,8.89
  Bottom 0.813: 77.47,12.06 v74.3,8.89 | 77.47,12.06 OUT_1.1 | CH0-2.1 79.5,14.09 77.47,12.06
  Bottom 1.27: v67.94,8.89 Q1.D | v74.3,8.89 74.3,9.53 75.56,10.79 | 76.83,12.06 78.74,13.97 81.92,13.97 | 85.09,13.97 81.92,13.97 | 81.92,13.97 78.11,17.78 75.56,17.78 75.56,10.79 | 75.56,10.79 76.83,12.06 | 76.83,12.06 76.83,17.14 77.47,17.14 80.01,14.61 78.11,14.61 78.11,15.88
OUTPUT_1  (via drill 0.6)
  Top 0.813: v73.66,20.32 v67.94,20.32
  Bottom 0.813: CH0-2.2 81.24,19.09 80.01,20.32 | 67.94,21.59 67.31,22.86
  Bottom 1.27: 66.04,22.86 67.31,22.86 67.94,22.86 67.94,21.59 v67.94,20.32 66.04,22.86 | Q2.D 66.04,22.86 | v73.66,20.32 OUT_1.2 80.01,20.32 81.28,19.05 85.09,19.05
OUTPUT_2  (via drill 0.6)
  Top 0.813: v73.66,36.83 v67.94,36.83
  Bottom 0.813: 81.28,24.13 85.05,24.13 CH0-2.3
  Bottom 1.27: v73.66,36.83 73.66,24.13 74.93,22.86 OUT_1.3 80.01,22.86 81.28,24.13 85.09,24.13 | v67.94,36.83 Q3.D
OUTPUT_3  (via drill 0.6)
  Top 0.813: v67.94,49.53 v73.66,49.53
  Bottom 0.813: CH3-5.1 80.77,56 80.64,55.88
  Bottom 1.27: v73.66,49.53 74.3,49.53 77.47,52.7 | 77.47,52.7 80.64,55.88 | 80.64,55.88 81.92,55.88 | 81.92,55.88 85.72,55.88 | v67.94,49.53 66.67,50.8 Q4.D | OUT_2.1 77.47,59.05 | 77.47,52.7 77.47,53.98 | 77.47,56.52 77.47,59.05 | 77.47,59.05 78.11,59.69 81.92,55.88 | 80.64,55.88 80.01,55.88 79.38,56.52 79.38,57.78 78.11,59.05 78.11,58.42 80.01,56.52 77.47,53.98 | 77.47,53.98 77.47,54.61 | 77.47,55.88 77.47,56.52 | 77.47,56.52 78.11,57.15 78.11,56.52 78.74,55.88 78.74,54.61 v73.66,49.53 | v73.66,49.53 73.66,52.07 77.47,55.88 | 77.47,55.88 77.47,54.61 | 77.47,54.61 74.3,51.44
OUTPUT_4  (via drill 0.6)
  Top 0.813: v73.66,62.23 v67.94,62.23
  Bottom 0.813: CH3-5.2 82.51,61 81.28,62.23
  Bottom 1.27: v67.94,62.23 67.94,63.5 66.67,64.77 Q5.D | v73.66,62.23 OUT_2.2 81.28,62.23 82.55,60.96 85.09,60.96
OUTPUT_5  (via drill 0.6)
  Top 0.813: v67.94,75.56 v73.66,75.56
  Bottom 0.813: CH3-5.3 82.51,66 81.28,64.77 OUT_2.3 76.83,64.77
  Bottom 1.27: 85.09,66.04 82.55,66.04 81.28,64.77 76.83,64.77 74.93,64.77 73.66,66.04 v73.66,75.56 | v67.94,75.56 66.04,77.47 Q6.D
RAW_INPUT
  Bottom 0.813: RAW.2 10.16,7.66 10.79,8.29 10.79,12.06 | U$2.VIN 10.79,12.06 | 10.16,15.88 10.16,12.7 10.79,12.06 | 10.79,12.06 11.43,12.7 11.43,16.51 10.16,16.51
RX
  Bottom 0.813: SERIAL_IN.3 31.11,9.53 29.21,11.43 29.21,19.05 U$2.RX
SCL
  Bottom 0.813: I2C.3 12.06,57.78 16.51,53.34 16.51,31.75 U$2.A5
SDA_/_D0
  Bottom 0.813: 12.06,54.61 13.97,52.7 13.97,34.29 U$2.A4 SPI.3 | 12.06,54.61 10.79,55.88 | 10.79,55.88 9.53,57.15 I2C.4 | 12.06,54.61 12.06,55.24 11.43,55.88 10.79,55.88
SERIAL_VCC
  Bottom 0.813: SERIAL_IN.4 34.29,12.06 35.56,13.34 SERIAL_VCC_JUMPER1.2
TX_3,3V
  Bottom 0.813: SERIAL_IN.2 R20.1 R19.2
TX_5V
  Bottom 0.813: R19.1 20.95,9.53 21.59,10.16 21.59,12.7 25.4,16.51 U$2.TX
(copper drawn outside any net)
  shapes: Bottom area x2

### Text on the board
Bottom: +12V | GND | VCC | +12V | +12V | GND | 6ch+ Serial / PWM driver / Boór András / 2017 | I2C display | VCC GND SCL SDA | display | ch3 - ch5 | +12V | ISP-5 | TX RX VCC | ch0 - ch2 | RAW | Serial In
